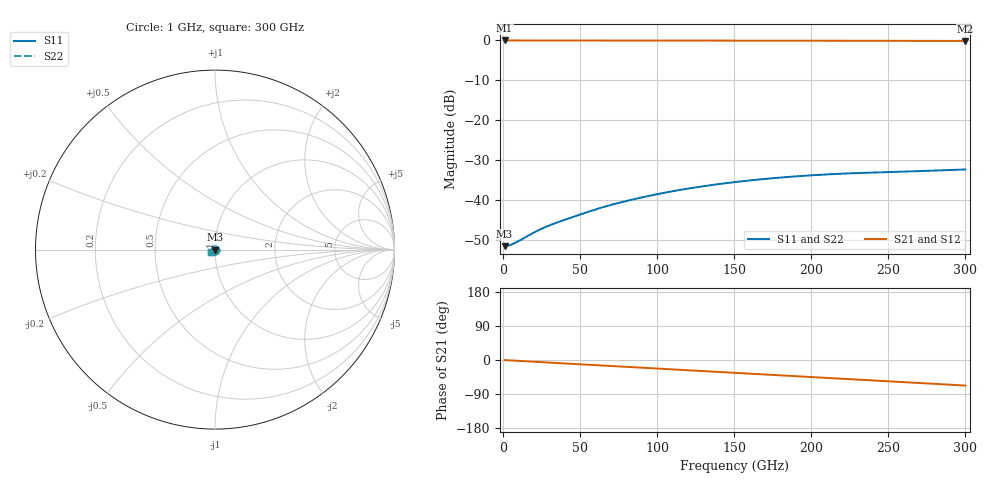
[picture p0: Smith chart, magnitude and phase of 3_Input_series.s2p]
#  Hz  S  RI  R  50
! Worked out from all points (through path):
!   300 points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, 1 GHz to 300 GHz, reference 50 ohm
!   highest |S21| = -0.02 dB at 1 GHz (marker M1); lowest = -0.1 dB at 300 GHz (marker M2)
!   group delay of S21, straight-line fit = 623 fs
!   lowest |S11| = -51.6 dB at 1 GHz (marker M3), VSWR 1.01, Z = 50.3 - j0.000586 ohm
!   |S11| at or under -10 dB: start of sweep to end of sweep
!   |S22| runs from -51.6 to -32.4 dB; largest |S21 - S12| = 0.00016
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1e9  0.00262 -5.83e-06  0.9974 -0.00406  0.9974 -0.00406  0.00262 -4.4e-06
4e9  0.00269 -3.45e-05  0.9972 -0.0162  0.9972 -0.0162  0.00269 -2.93e-05
7e9  0.00283 -0.000101  0.9967 -0.0283  0.9967 -0.0283  0.00283 -9.38e-05
1e10  0.00302 -0.000227  0.9961 -0.0403  0.9961 -0.0403  0.00303 -0.000219
2e10  0.00372 -0.00114  0.9928 -0.0796  0.9928 -0.0796  0.00373 -0.00114
2.8e10  0.00403 -0.00221  0.9895 -0.1107  0.9895 -0.1107  0.00403 -0.00222
3.6e10  0.0041 -0.00332  0.9852 -0.1417  0.9852 -0.1417  0.0041 -0.00332
5.1e10  0.00396 -0.00534  0.9745 -0.1993  0.9744 -0.1993  0.00396 -0.00534
6.2e10  0.00363 -0.00689  0.9646 -0.2409  0.9646 -0.2409  0.00363 -0.0069
7.3e10  0.00305 -0.00841  0.953 -0.2821  0.953 -0.2821  0.00305 -0.00841
8.7e10  0.00208 -0.0102  0.9357 -0.3337  0.9357 -0.3336  0.00209 -0.0102
1.01e11  0.000874 -0.0119  0.9157 -0.3842  0.9157 -0.3842  0.000873 -0.0119
1.12e11  -0.000257 -0.013  0.898 -0.4231  0.898 -0.4231  -0.000258 -0.013
1.25e11  -0.00173 -0.0142  0.875 -0.468  0.875 -0.468  -0.00173 -0.0142
1.38e11  -0.00332 -0.0152  0.8499 -0.5117  0.8499 -0.5117  -0.00333 -0.0152
1.51e11  -0.00503 -0.016  0.8225 -0.5541  0.8225 -0.5541  -0.00503 -0.016
1.76e11  -0.00839 -0.0168  0.7639 -0.6314  0.7639 -0.6314  -0.0084 -0.0168
2.01e11  -0.0117 -0.0167  0.6979 -0.7025  0.6979 -0.7025  -0.0117 -0.0167
2.24e11  -0.0143 -0.016  0.631 -0.762  0.631 -0.762  -0.0143 -0.016
2.51e11  -0.0167 -0.0147  0.5459 -0.8233  0.5459 -0.8233  -0.0167 -0.0147
2.78e11  -0.0188 -0.0136  0.4554 -0.8742  0.4554 -0.8743  -0.0189 -0.0136
3e11  -0.0206 -0.0124  0.378 -0.9085  0.3781 -0.9083  -0.0206 -0.0124
